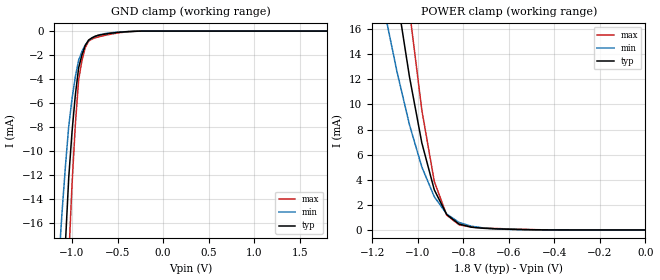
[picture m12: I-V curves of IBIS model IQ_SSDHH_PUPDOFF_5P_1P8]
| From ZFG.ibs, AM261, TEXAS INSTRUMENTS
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[Model]   IQ_SSDHH_PUPDOFF_5P_1P8
Model_type   Input
Polarity   Non-Inverting
Vinl =  0.63
Vinh =  1.17
C_comp   1.313442p   1.241204p   1.780255p
|[Input load] weak_pupdoff
|[supplytol] 5
|[temp] ind
[Model Spec]
Vinl   0.63   0.5985   0.6615
Vinh   1.17   1.1115   1.2285
[Temperature Range]   25   125   -40
[Voltage Range]   1.8   1.71   1.89
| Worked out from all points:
|   GND clamp passes 1 mA (typ) near -0.84 V on its own axis
|   POWER clamp passes 1 mA (typ) near -0.86 V on its own axis
| Nom Voltages:
|   VDD=1.1, VDDS=1.8, VDDS18=1.8, BUS_VSSS=0, ESD_BIASFET=0, VSS=0
| Min Voltages:
|   VDD=1.045, VDDS=1.71, VDDS18=1.71, BUS_VSSS=0, ESD_BIASFET=0, VSS=0
| Max Voltages:
|   VDD=1.16, VDDS=1.89, VDDS18=1.89, BUS_VSSS=0, ESD_BIASFET=0, VSS=0
[POWER_clamp]
|   voltage   I(typ)   I(min)   I(max)
-1.8V     125.7mA    90.95mA    174.2mA
-1.127V   23.26mA    15.8mA     33.5mA
-1.073V   16.45mA    11.19mA    23.69mA
-1.055V   14.33mA    9.791mA    20.59mA
-1.036V   12.21mA    8.39mA     17.49mA
-1.018V   10.45mA    7.264mA    14.84mA
-981.8mV  6.927mA    5.012mA    9.53mA
-927.3mV  3.2mA      2.646mA    3.869mA
-872.7mV  1.228mA    1.269mA    1.178mA
-818.2mV  468.1uA    595.3uA    409.5uA
-654.5mV  88.28uA    84.44uA    116.7uA
0V        19.84nA    103.8nA    217.5nA
[GND_clamp]
|   voltage   I(typ)   I(min)   I(max)
-1.8V     -190.2mA   -126mA     -287.6mA
-1.145V   -30.71mA   -19.26mA   -48.24mA
-1.109V   -23.91mA   -15.06mA   -37.5mA
-1.073V   -17.75mA   -11.29mA   -27.75mA
-1.036V   -12.24mA   -7.958mA   -18.98mA
-1V       -8.39mA    -5.645mA   -12.77mA
-963.6mV  -5.329mA   -3.799mA   -7.793mA
-927.3mV  -3.057mA   -2.421mA   -4.049mA
-854.5mV  -1.206mA   -1.153mA   -1.368mA
-781.8mV  -563.5uA   -592.1uA   -675.2uA
-272.7mV  -6.512uA   -13.21uA   -7.453uA
1.8V      19.84nA    106.3nA    209.3nA
